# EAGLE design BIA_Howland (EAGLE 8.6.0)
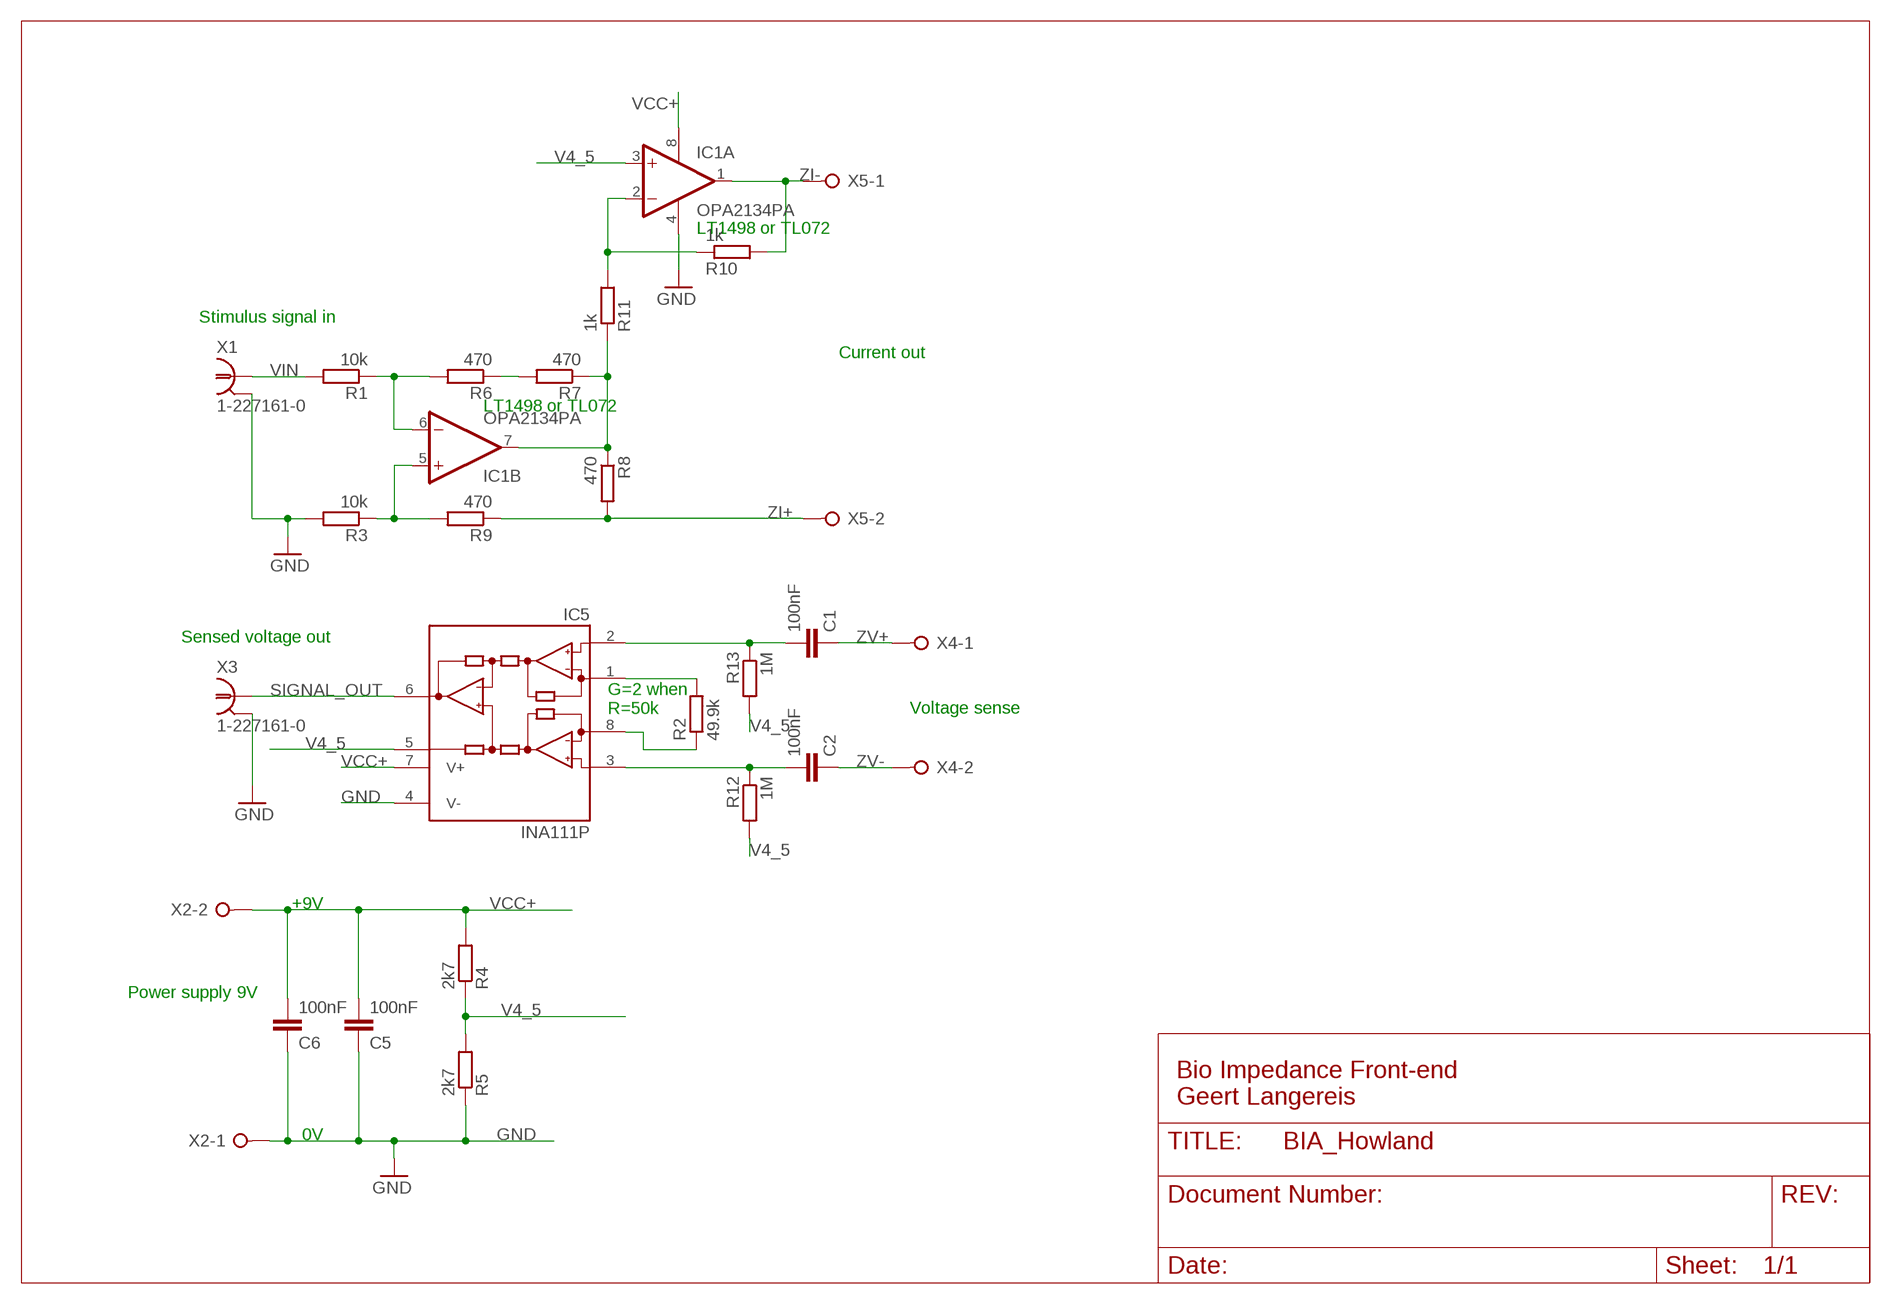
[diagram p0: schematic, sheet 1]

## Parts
C1  100nF  C-EU050-025X075  [C050-025X075]
C2  100nF  C-EU050-025X075  [C050-025X075]
C5  100nF  C-EU050-025X075  [C050-025X075]
C6  100nF  C-EU050-025X075  [C050-025X075]
IC1  OPA2134PA  [DIL08]
IC5  INA111P  [DIL08]
R1  10k  R-EU_0204/7  [0204/7]
R2  49.9k  R-EU_0204/7  [0204/7]
R3  10k  R-EU_0204/7  [0204/7]
R4  2k7  R-EU_0204/7  [0204/7]
R5  2k7  R-EU_0204/7  [0204/7]
R6  470  R-EU_0204/7  [0204/7]
R7  470  R-EU_0204/7  [0204/7]
R8  470  R-EU_0204/7  [0204/7]
R9  470  R-EU_0204/7  [0204/7]
R10  1k  R-EU_0204/7  [0204/7]
R11  1k  R-EU_0204/7  [0204/7]
R12  1M  R-EU_0204/7  [0204/7]
R13  1M  R-EU_0204/7  [0204/7]
X1  1-227161-0  [AMP_227161]
X2  W237-02P  [W237-132]
X3  1-227161-0  [AMP_227161]
X4  W237-02P  [W237-132]
X5  W237-02P  [W237-132]

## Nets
GND: C5.1 C6.1 IC1.4(A:V-) IC5.4(V-) R3.2 R5.1 X1.2 X2.1 X3.2
N$1: C1.2 IC5.2(-IN) R13.1
N$2: IC1.5(B:+IN) R3.1 R9.2
N$3: IC5.1(RG) R2.2
N$4: IC5.8(RG) R2.1
N$5: C2.2 IC5.3(+IN) R12.1
N$6: IC1.7(B:OUT) R7.1 R8.1 R11.1
N$7: R6.1 R7.2
N$8: IC1.6(B:-IN) R1.1 R6.2
N$12: IC1.2(A:-IN) R10.1 R11.2
SIGNAL_OUT: IC5.6(OUT) X3.1
V4_5: IC1.3(A:+IN) IC5.5(REF) R4.1 R5.2 R12.2 R13.2
VCC+: C5.2 C6.2 IC1.8(A:V+) IC5.7(V+) R4.2 X2.2
VIN: R1.2 X1.1
ZI+: R8.2 R9.1 X5.2
ZI-: IC1.1(A:OUT) R10.2 X5.1
ZV+: C1.1 X4.1
ZV-: C2.1 X4.2

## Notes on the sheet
- LT1498 or TL072
- Stimulus signal in
- Current out
- LT1498 or TL072
- Sensed voltage out
- G=2 when 
  R=50k
- Voltage sense
- +9V
- Power supply 9V
- Bio Impedance Front-end
  Geert Langereis
- 0V

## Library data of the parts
C1 C2 C5 C6 = rcl:C-EU: CAPACITOR, European symbol
IC1 = linear:OPA2*: Dual Operational Amplifier Low Power, Single-Supply, Rail-To-Rail Operational Amplifier Source: http://focus.ti.com/lit/ds/symlink/opa2345.pdf http://focus.ti.com .. opa241.pdf http://focus.ti.com/lit/ds/symlink/opa2134.pdf
IC5 = burr-brown:INA111: Instrumentation Amplifier High Speed FET-Input; MF: TEXAS INSTRUMENT CONNECTORS; MPN: INA111BP; OC_FARNELL: 1212397; OC_NEWARK: 27C4351
R1-R13 = rcl:R-EU_: RESISTOR, European symbol
X1 X3 = con-coax:?227161*: JACK, RIGHT ANGLE, 50 OHM, PCB, BNC; MF: TYCO ELECTRONICS; MPN: 1-227161; OC_FARNELL: unknown; OC_NEWARK: 33B3200
X2 X4 X5 = con-wago-508:W237-02P: WAGO SREW CLAMP; OC_FARNELL: unknown; OC_NEWARK: unknown

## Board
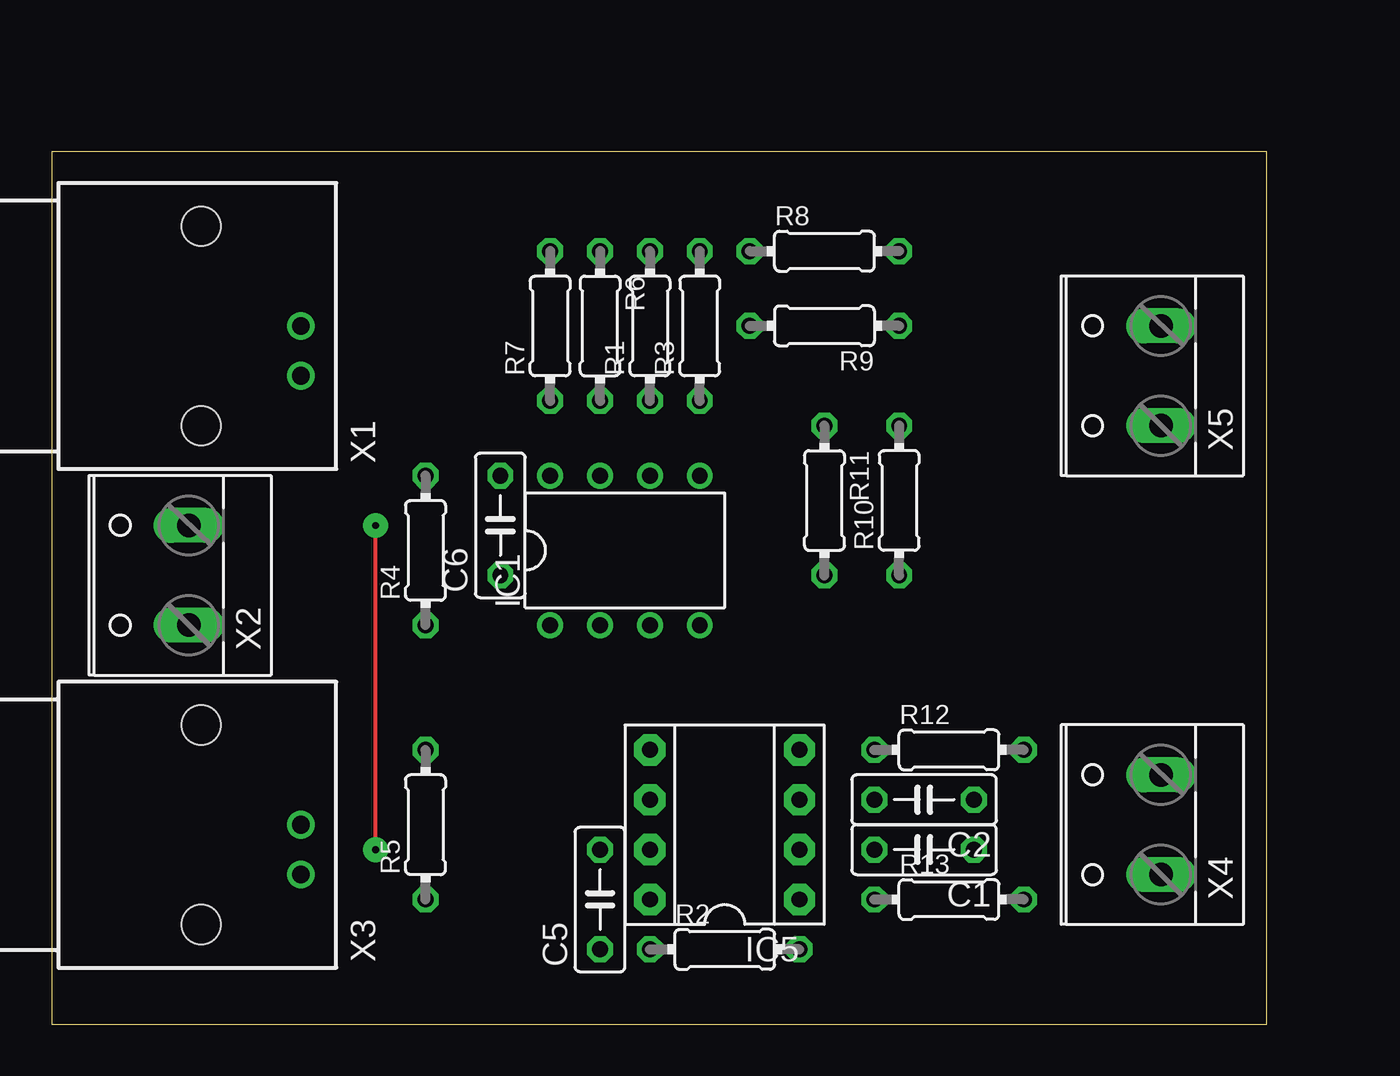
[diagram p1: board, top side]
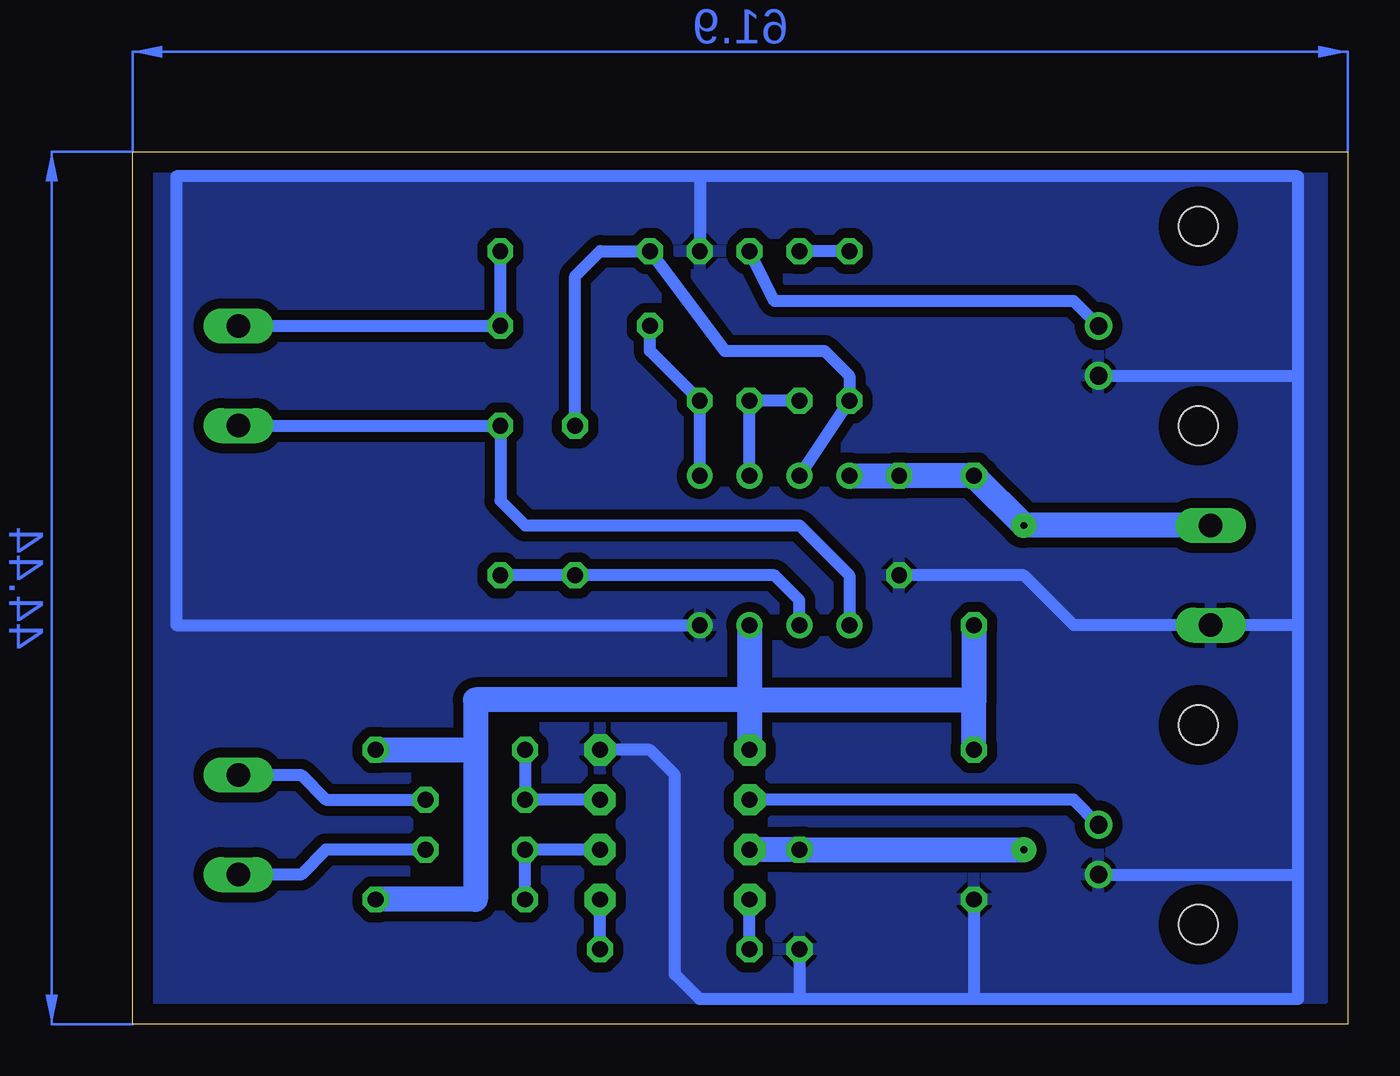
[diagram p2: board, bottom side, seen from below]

Size 61.9 x 44.44 mm. Coordinates in mm from the lower left corner, seen from the top.
Outline: 0,0 61.9,0 61.9,44.44 0,44.44 0,0
Copper layers (1*16): Top 0.035mm / dielectric 1.5mm / Bottom 0.035mm
Design rules "default *": minimum track width 6mil, minimum drill 0.35mm, track to track 20mil, track to pad 20mil, pad to pad 20mil, via to via 20mil, smd to smd 6mil, copper to edge 40mil, drill to drill 6mil, minimum pad ring 10mil, minimum via ring 18mil, stop-mask expansion 4mil, vias tented up to drill 0mil, thermal gap 10mil

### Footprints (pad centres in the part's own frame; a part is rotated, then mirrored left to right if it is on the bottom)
C050-025X075 = drill 0.813 octagon: 1 -2.54,0; 2 2.54,0
DIL08 = drill 0.813 pad 1.27: 1 -3.81,-3.81; 2 -1.27,-3.81; 3 1.27,-3.81; 4 3.81,-3.81; 5 3.81,3.81; 6 1.27,3.81; 7 -1.27,3.81; 8 -3.81,3.81
DIL08' = drill 0.813 pad 1.6 octagon: 1 -3.81,-3.81; 2 -1.27,-3.81; 3 1.27,-3.81; 4 3.81,-3.81; 5 3.81,3.81; 6 1.27,3.81; 7 -1.27,3.81; 8 -3.81,3.81
0204/7 = drill 0.813 octagon: 1 -3.81,0; 2 3.81,0
AMP_227161 = drill 0.9 pad 1.27: 1 0,-5.08; 2 -2.54,-5.08 | hole 2: -5.08,0; 5.08,0
W237-132 = drill 1.194 long: 1 -2.54,-0.635; 2 2.54,-0.635

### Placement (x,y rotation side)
C1  44.45,8.89 180 top
C2  44.45,11.43 180 top
C5  27.94,6.35 90 top
C6  22.86,25.4 90 top
IC1  29.21,24.13 0 top
IC5  INA111P  [DIL08']  34.29,10.16 90 top
R1  30.48,35.56 90 top
R2  34.29,3.81 0 top
R3  33.02,35.56 90 top
R4  19.05,24.13 90 top
R5  19.05,10.16 90 top
R6  27.94,35.56 270 top
R7  25.4,35.56 90 top
R8  39.37,39.37 0 top
R9  39.37,35.56 180 top
R10  43.18,26.67 90 top
R11  39.37,26.67 270 top
R12  45.72,13.97 0 top
R13  45.72,6.35 0 top
X1  7.62,35.56 90 top
X2  6.35,22.86 90 top
X3  7.62,10.16 90 top
X4  55.88,10.16 90 top
X5  55.88,33.02 90 top

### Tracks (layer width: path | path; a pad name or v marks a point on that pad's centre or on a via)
GND
  Bottom 0.61: C6.1 16.51,22.86 13.97,20.32 X2.1 2.54,20.32 | 2.54,33.02 2.54,43.18 33.02,43.18 | 2.54,33.02 2.54,20.32 | 2.54,20.32 2.54,7.62 | 2.54,7.62 2.54,1.27 19.05,1.27 | 33.02,43.18 R3.2 | 19.05,1.27 27.94,1.27 | 27.94,1.27 33.02,1.27 34.29,2.54 34.29,12.7 35.56,13.97 IC5.4 | R5.1 19.05,1.27 | C5.1 27.94,1.27 | 33.02,43.18 59.69,43.18 59.69,20.32 IC1.4 | X1.2 2.54,33.02 | X3.2 2.54,7.62
  pour Bottom: 1.27,43.18 60.96,43.18 60.96,1.27 1.27,1.27
N$1
  Bottom 0.61: IC5.2 C1.2 R13.1
N$2
  Bottom 0.61: IC1.5 R3.1 35.56,34.29 R9.2
N$3
  Bottom 0.61: R2.2 IC5.1
N$4
  Bottom 0.61: R2.1 IC5.8
N$5
  Bottom 0.61: IC5.3 C2.2 R12.1
N$6
  Bottom 0.61: IC1.7 R7.1 25.4,33.02 26.67,34.29 31.75,34.29 R8.1 38.1,39.37 39.37,38.1 R11.1
N$7
  Bottom 0.61: R7.2 R6.1
N$8
  Bottom 0.61: IC1.6 R1.1 R6.2
N$12
  Bottom 0.61: IC1.2 27.94,21.59 29.21,22.86 R11.2 R10.1
SIGNAL_OUT
  Bottom 0.61: X3.1 13.97,11.43 IC5.6
V4_5
  Bottom 1.27: R4.1 19.05,16.51 | R5.2 19.05,16.51 | 30.48,16.51 19.05,16.51 | 30.48,16.51 IC5.5 | IC1.3 30.48,16.51 | 30.48,16.51 44.45,16.51 44.45,13.97 | 44.45,13.97 44.45,6.35 R13.2 | R12.2 44.45,13.97
VCC+  (via drill 0.35)
  Top 0.203: v16.51,8.89 v16.51,25.4
  Bottom 1.27: IC5.7 C5.2 v16.51,8.89 | X2.2 v16.51,25.4 R4.2 C6.2 IC1.8
VIN
  Bottom 0.61: X1.1 13.97,36.83 29.21,36.83 R1.2
ZI+
  Bottom 0.61: R8.2 R9.1 X5.2
ZI-
  Bottom 0.61: IC1.1 25.4,22.86 27.94,25.4 41.91,25.4 43.18,26.67 R10.2 X5.1
ZV+
  Bottom 0.61: C1.1 52.07,8.89 53.34,7.62 X4.1
ZV-
  Bottom 0.61: X4.2 53.34,12.7 52.07,11.43 C2.1
(copper drawn outside any net)
  shapes: Bottom area x2

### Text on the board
bRestrict: Geert Langereis, / January 2018 / BIA Interface v2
